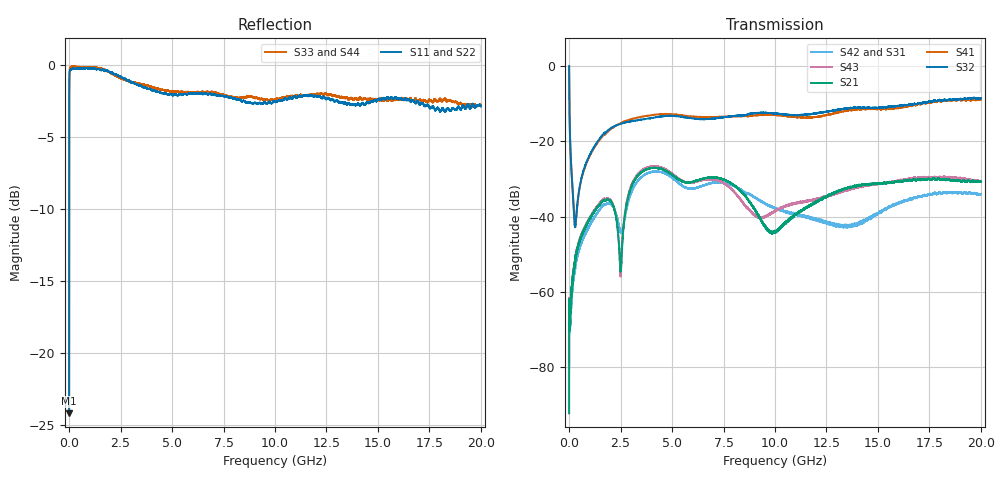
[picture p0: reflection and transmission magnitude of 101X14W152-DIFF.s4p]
!{101X14W152}
!Johanson Technology Inc.
!www.johansontechnology.com
!Test Board Conditions:
!Substrate Type  RO4350B
!Substrate Thickness  10 mil
!Substrate Dk  3.66
!TL Type: GCPW
!TL Trace Width  20 mil
!TL Gap  15 mil
!PART MODE DIFFERENTIAL
!DUT TOPOLOGY	DIFFERENTIAL 4-PORT
!Mounting Pad LxW  20x35 mil
# MHz S  dB  R 50
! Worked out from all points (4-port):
!   20001 points, 300 kHz to 20 GHz, reference 50 ohm
!   strongest paths, dB at 300 kHz, 5 GHz, 10 GHz, 15 GHz, 20 GHz:
!     S32: 0.0, -13.2, -12.6, -11.1, -8.5
!     S41: -0.1, -12.8, -13.0, -11.4, -8.9
!     S21: -92.3, -28.9, -43.9, -31.2, -30.7
!     S43: -79.2, -28.6, -38.6, -31.3, -30.6
!     S42: -81.1, -29.7, -37.7, -39.3, -34.1
!     S31: -76.4, -29.6, -37.7, -39.2, -34.2
!   lowest |S11| = -24.2 dB at 300 kHz (marker M1), VSWR 1.13, Z = 49.8 - j6.16 ohm
!   |S11| at or under -10 dB: start of sweep to 1.773 MHz
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0.3  -24.21 -88.1  -76.77 116.1  -78.04 -161.9  -0.07 -3.8
     -92.29 170.6  -24.16 -94.2  -0.03 -3.6  -83.66 4.4
     -76.40 120.0  -0.02 -3.4  -24.03 -93.4  -77.09 115.9
     -0.08 -3.8  -81.10 122.0  -79.17 -111.4  -24.08 -87.7
309.295  -0.25 178.5  -51.17 78.8  -52.61 78.6  -41.92 9.2
         -50.66 78.8  -0.17 177.7  -41.96 11.8  -52.49 74.9
         -52.62 75.7  -41.93 11.7  -0.10 177.5  -50.47 78.6
         -41.96 8.7  -52.78 75.8  -50.60 77.8  -0.07 177.3
1792.273  -0.36 164.6  -35.62 37.4  -36.67 28.4  -17.87 60.7
          -35.67 36.8  -0.39 164.0  -17.59 58.3  -36.71 28.2
          -36.67 28.1  -17.58 58.3  -0.35 163.0  -35.30 36.3
          -17.93 60.7  -36.69 27.9  -35.32 36.4  -0.31 163.5
2506.262  -0.77 161.2  -54.06 -121.2  -44.04 -108.7  -15.15 45.6
          -54.23 -121.8  -0.86 160.8  -15.37 40.7  -44.13 -109.8
          -43.97 -109.5  -15.35 40.7  -0.88 159.0  -55.55 -132.0
          -15.15 45.7  -44.26 -110.0  -55.70 -130.7  -0.82 159.2
3766.244  -1.59 155.5  -27.41 55.4  -28.53 50.7  -13.20 25.9
          -27.45 55.6  -1.34 157.8  -14.01 25.3  -28.58 51.2
          -28.59 50.8  -13.99 25.2  -1.38 154.1  -26.96 52.8
          -13.24 26.0  -28.57 51.2  -26.97 52.8  -1.48 153.2
9882.152  -2.58 127.0  -44.27 -11.2  -37.59 -69.9  -12.98 -11.9
          -44.25 -12.3  -2.32 125.3  -12.59 -9.5  -37.61 -70.0
          -37.51 -70.0  -12.54 -10.0  -2.40 120.5  -38.85 5.9
          -13.00 -12.1  -37.47 -70.3  -38.87 6.4  -2.48 124.7
20000  -2.85 76.6  -30.81 -36.1  -34.29 -85.0  -8.91 -40.9
       -30.71 -35.7  -3.13 75.9  -8.49 -45.3  -33.96 -83.1
       -34.21 -84.5  -8.49 -44.3  -2.77 59.6  -30.49 -49.3
       -8.93 -40.3  -34.06 -82.6  -30.55 -49.6  -2.53 64.3
